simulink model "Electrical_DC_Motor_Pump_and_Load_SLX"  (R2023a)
settings: Solver=ode23s  StartTime=0.0  StopTime=10.0  MaxStep=0.001  RelTol=1e-3
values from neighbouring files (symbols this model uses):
  b_7 = 0.1*Nm/(rad/sec)    (= 0.1)    [Electrical_DC_Motor_Pump_and_Load_EQN.m]    (also in Electrical_DC_Motor_Pump_and_Load_SLX_m.m; Car_Dumper_EQN.m = 2; Car_Dumper_SLX_m.m = 2; Electrical_DC_Motor_EQN.m)
  C_b = 0.001*m^3/Pa    (= 0.001)    [Electrical_DC_Motor_Pump_and_Load_EQN.m]    (also in Electrical_DC_Motor_Pump_and_Load_SLX_m.m; Electrical_DC_Motor_and_Pump_EQN.m; Electrical_DC_Motor_and_Pump_SLX_m.m)
  I_2_0 = 0*A    (= 0)    [Electrical_DC_Motor_Pump_and_Load_SLX_m.m]    (also in Electric_Circuit_02_SLX_m.m; Electric_Circuit_03_SLX_m.m; Electric_Circuit_06_SLX_m.m; Electric_Circuit_08_SLX_m.m)
  J_6 = 0.01*kg*m^2    (= 0.01)    [Electrical_DC_Motor_Pump_and_Load_EQN.m]    (also in Electrical_DC_Motor_Pump_and_Load_SLX_m.m; Electrical_DC_Motor_EQN.m; Electrical_DC_Motor_SLX_m.m; Electrical_DC_Motor_and_Pump_EQN.m)
  K_q = 1    [Electrical_DC_Motor_Pump_and_Load_EQN.m]    (also in Electrical_DC_Motor_Pump_and_Load_SLX_m.m; Electrical_DC_Motor_and_Pump_EQN.m; Electrical_DC_Motor_and_Pump_SLX_m.m)
  K_t = 1    [Electrical_DC_Motor_Pump_and_Load_EQN.m]    (also in Electrical_DC_Motor_Pump_and_Load_SLX_m.m; Electrical_DC_Motor_and_Pump_EQN.m; Electrical_DC_Motor_and_Pump_SLX_m.m)
  L_2 = 0.002*H    (= 0.002)    [Electrical_DC_Motor_Pump_and_Load_EQN.m]    (also in Electrical_DC_Motor_Pump_and_Load_SLX_m.m; Electric_Circuit_02_EQN.m; Electric_Circuit_02_SLX_m.m; Electric_Circuit_03_EQN.m)
  L_d = 10*Pa*sec^2/m^3    (= 10)    [Electrical_DC_Motor_Pump_and_Load_EQN.m]    (also in Electrical_DC_Motor_Pump_and_Load_SLX_m.m)
  P_b_0 = 0*Pa    (= 0)    [Electrical_DC_Motor_Pump_and_Load_SLX_m.m]    (also in Electrical_DC_Motor_and_Pump_SLX_m.m)
  Q_d_0 = 0*m^3/sec    (= 0)    [Electrical_DC_Motor_Pump_and_Load_SLX_m.m]    (also in Electrical_DC_Motor_and_Pump_SLX_m.m)
  Q_g_0 = 0*m^3/sec    (= 0)    [Electrical_DC_Motor_Pump_and_Load_SLX_m.m]
  R_3 = 100*Ohm    (= 100)    [Electrical_DC_Motor_Pump_and_Load_EQN.m]    (also in Electrical_DC_Motor_Pump_and_Load_SLX_m.m; Electric_Circuit_01_EQN.m; Electric_Circuit_01_SLX_m.m; Electric_Circuit_02_EQN.m)
  R_c = 10000*Pa/(m^3/sec)    (= 10000)    [Electrical_DC_Motor_Pump_and_Load_EQN.m]    (also in Electrical_DC_Motor_Pump_and_Load_SLX_m.m; Electrical_DC_Motor_and_Pump_EQN.m; Electrical_DC_Motor_and_Pump_SLX_m.m)
  R_e = 10000*Pa/(m^3/sec)    (= 10000)    [Electrical_DC_Motor_Pump_and_Load_EQN.m]    (also in Electrical_DC_Motor_Pump_and_Load_SLX_m.m)
  R_f = 10000*Pa/(m^3/sec)    (= 10000)    [Electrical_DC_Motor_Pump_and_Load_EQN.m]    (also in Electrical_DC_Motor_Pump_and_Load_SLX_m.m; BIG_EC_Simscape_EQN.m = 100; BIG_EC_Simscape_SLX_m.m = 100)
  Ts = Tfin/Nr_Ts_Points    (= 0.00054055)    [Electrical_DC_Motor_Pump_and_Load_SLX_m.m]    (also in BIG_EC_Simscape_SLX_m.m = 0.0003; Car_Dumper_SLX_m.m = 0.0022779; Electric_Circuit_01_SLX_m.m = 0.005; Electric_Circuit_02_SLX_m.m = 0.000480145)
  V_1_0 = 10*V    (= 10)    [Electrical_DC_Motor_Pump_and_Load_SLX_m.m]    (also in BIG_EC_Simscape_SLX_m.m; Electric_Circuit_02_SLX_m.m; Electric_Circuit_03_SLX_m.m; Electric_Circuit_04_SLX_m.m)
  w_6_0 = 0*rad/sec    (= 0)    [Electrical_DC_Motor_Pump_and_Load_SLX_m.m]    (also in Electrical_DC_Motor_SLX_m.m; Electrical_DC_Motor_and_Pump_SLX_m.m)

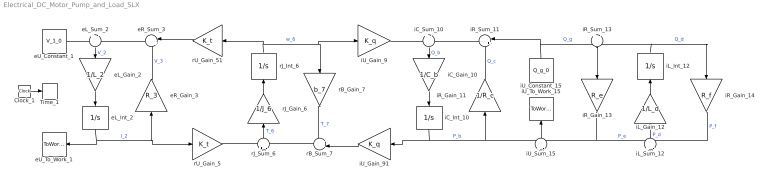
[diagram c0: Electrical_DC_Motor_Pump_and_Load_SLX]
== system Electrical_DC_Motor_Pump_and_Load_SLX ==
  Clock_1 : Clock
  Time_1 : ToWorkspace  VariableName=t  SaveFormat=Timeseries  SampleTime=Ts
  eL_Gain_2 : Gain  Gain=1/L_2  Multiplication=Matrix(K*u)
  eL_Int_2 : Integrator  InitialCondition=I_2_0
  eL_Sum_2 : Sum  Inputs=+|-
  eR_Gain_3 : Gain  Gain=R_3  Multiplication=Matrix(K*u)
  eR_Sum_3 : Sum  Inputs=|++
  eU_Constant_1 : Constant  Value=V_1_0
  eU_To_Work_1 : ToWorkspace  VariableName=I_1_0  SaveFormat=Timeseries  SampleTime=Ts
  iC_Gain_10 : Gain  Gain=1/C_b  Multiplication=Matrix(K*u)
  iC_Int_10 : Integrator  InitialCondition=P_b_0
  iC_Sum_10 : Sum  Inputs=+|-
  iL_Gain_12 : Gain  Gain=1/L_d  Multiplication=Matrix(K*u)
  iL_Int_12 : Integrator  InitialCondition=Q_d_0
  iL_Sum_12 : Sum  Inputs=+|-
  iR_Gain_11 : Gain  Gain=1/R_c  Multiplication=Matrix(K*u)
  iR_Gain_13 : Gain  Gain=R_e  Multiplication=Matrix(K*u)
  iR_Gain_14 : Gain  Gain=R_f  Multiplication=Matrix(K*u)
  iR_Sum_11 : Sum  Inputs=|++
  iR_Sum_13 : Sum  Inputs=+|-
  iU_Constant_15 : Constant  Value=Q_g_0
  iU_Gain_9 : Gain  Gain=K_q  Multiplication=Matrix(K*u)
  iU_Gain_91 : Gain  Gain=K_q  Multiplication=Matrix(K*u)
  iU_Sum_15 : Sum  Inputs=+|-
  iU_To_Work_15 : ToWorkspace  VariableName=P_g_0  SaveFormat=Timeseries  SampleTime=Ts
  rB_Gain_7 : Gain  Gain=b_7  Multiplication=Matrix(K*u)
  rB_Sum_7 : Sum  Inputs=++|
  rJ_Gain_6 : Gain  Gain=1/J_6  Multiplication=Matrix(K*u)
  rJ_Int_6 : Integrator  InitialCondition=w_6_0
  rJ_Sum_6 : Sum  Inputs=+|-
  rU_Gain_5 : Gain  Gain=K_t  Multiplication=Matrix(K*u)
  rU_Gain_51 : Gain  Gain=K_t  Multiplication=Matrix(K*u)
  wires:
  eU_Constant_1/1 -> eL_Sum_2/1
  eR_Sum_3/1 -> eL_Sum_2/2
  eL_Int_2/1 -> eU_To_Work_1/1, eR_Gain_3/1, rU_Gain_5/1  "I_2"
  eL_Sum_2/1 -> eL_Gain_2/1  "V_2"
  eL_Gain_2/1 -> eL_Int_2/1
  rU_Gain_51/1 -> eR_Sum_3/1
  eR_Gain_3/1 -> eR_Sum_3/2  "V_3"
  rU_Gain_5/1 -> rJ_Sum_6/1
  rJ_Int_6/1 -> rU_Gain_51/1, rB_Gain_7/1, iU_Gain_9/1  "w_6"
  rB_Sum_7/1 -> rJ_Sum_6/2
  rJ_Sum_6/1 -> rJ_Gain_6/1  "T_6"
  rJ_Gain_6/1 -> rJ_Int_6/1
  iU_Gain_91/1 -> rB_Sum_7/2
  rB_Gain_7/1 -> rB_Sum_7/1  "T_7"
  iU_Gain_9/1 -> iC_Sum_10/1
  iC_Int_10/1 -> iU_Gain_91/1, iR_Gain_11/1, iU_Sum_15/1  "P_b"
  iR_Sum_11/1 -> iC_Sum_10/2
  iC_Sum_10/1 -> iC_Gain_10/1  "Q_b"
  iC_Gain_10/1 -> iC_Int_10/1
  iU_Constant_15/1 -> iR_Sum_11/1, iR_Sum_13/1  "Q_g"
  iR_Gain_11/1 -> iR_Sum_11/2  "Q_c"
  iR_Gain_13/1 -> iU_Sum_15/2, iL_Sum_12/1  "P_e"
  iU_Sum_15/1 -> iU_To_Work_15/1
  iL_Int_12/1 -> iR_Sum_13/2, iR_Gain_14/1  "Q_d"
  iR_Sum_13/1 -> iR_Gain_13/1
  iR_Gain_14/1 -> iL_Sum_12/2  "P_f"
  iL_Sum_12/1 -> iL_Gain_12/1  "P_d"
  iL_Gain_12/1 -> iL_Int_12/1
  Clock_1/1 -> Time_1/1
